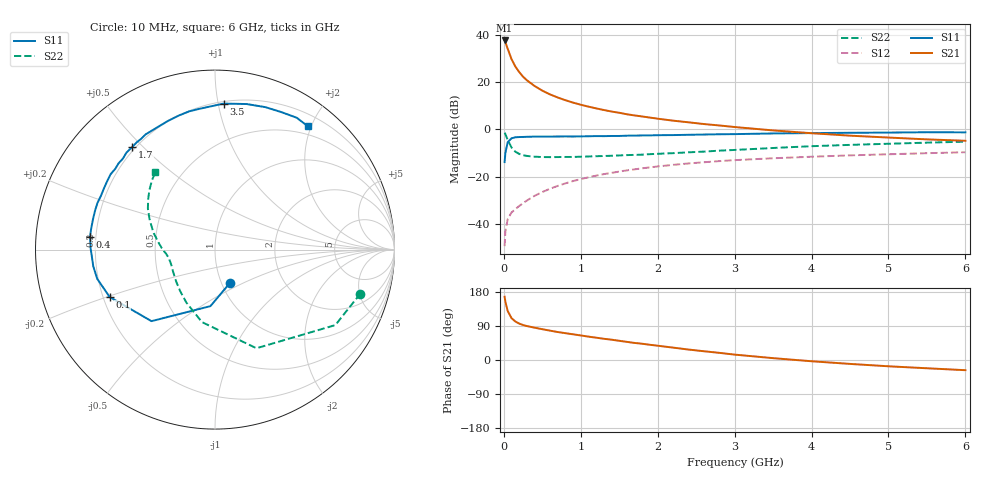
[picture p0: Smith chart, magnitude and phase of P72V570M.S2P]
! SIEMENS Small Signal Semiconductors
! BFP196
! Si NPN RF Bipolar Junction Transistor in SOT143
! VCE = 2.5 V  IC = 70 mA
! Common Emitter S-Parameters:  May  1996
# GHz  S  MA  R  50
!  f  S11  S21  S12  S22
! GHz  MAG  ANG  MAG  ANG  MAG  ANG  MAG  ANG
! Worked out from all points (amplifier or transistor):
!   36 points, 10 MHz to 6 GHz, reference 50 ohm
!   highest |S21| = 37.5 dB at 10 MHz (marker M1)
!   |S21| within 3 dB of that: start of sweep to 44.55 MHz
!   unconditionally stable (mu >= 1): 373.3 MHz to 4.492 GHz
!   at 250 MHz: K = 0.92, MSG = 26.7 dB, |S12| = -31.2 dB
!   at 1.4 GHz: K = 1.09, MAG = 11.1 dB, |S12| = -18.4 dB
!   at 6 GHz: K = 0.99, MSG = 2.4 dB, |S12| = -9.7 dB
!   S11 on the Smith chart (normalised r, x): 10 MHz: 1.10, -0.42; 100 MHz: 0.23, -0.20; 400 MHz: 0.18, +0.05; 1.7 GHz: 0.19, +0.46; 3.5 GHz: 0.21, +1.04; 6 GHz: 0.37, +1.95
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0.01  0.2024 -65.2  74.92 166.9  0.0034 77.6  0.8465 -16.8
0.02  0.3159 -94.6  69.35 153.9  0.007 69.7  0.7914 -32.1
0.05  0.5331 -131.6  49.97 129.3  0.0126 54.3  0.5962 -67.2
0.1  0.6437 -155.8  30.19 110.4  0.0175 49.4  0.4104 -100.2
0.15  0.6761 -166.1  21.05 101.5  0.0206 52.5  0.3354 -118.4
0.2  0.6846 -172.2  16.09 96.1  0.024 56.1  0.3014 -130.2
0.25  0.6876 -177.1  12.86 92.3  0.0274 58.2  0.2828 -138.9
0.3  0.6925 179.8  10.8 89.6  0.0313 61.3  0.2734 -144.6
0.4  0.6996 174.1  8.169 85.2  0.0394 63.8  0.2633 -152.9
0.5  0.6998 170.2  6.53 81.3  0.0472 64.8  0.2588 -158.4
0.6  0.7007 165.7  5.445 77.5  0.0555 65.0  0.2579 -162.1
0.7  0.7028 161.7  4.684 73.8  0.0636 65.2  0.2586 -164.7
0.9  0.7027 154.7  3.649 67.8  0.0806 63.4  0.2601 -169.1
1.1  0.7113 147.7  3.003 61.7  0.0966 61.5  0.2664 -172.0
1.3  0.7152 141.0  2.547 56.0  0.1129 58.9  0.2725 -174.8
1.7  0.7345 129.0  1.956 45.0  0.1424 53.1  0.2876 -179.8
2.2  0.7529 115.7  1.518 32.7  0.1771 45.6  0.3128 174.0
3  0.7893 96.2  1.114 14.2  0.2227 33.4  0.3656 162.2
3.5  0.815 86.6  0.945 4.9  0.2441 26.4  0.4021 155.1
4.5  0.8419 70.5  0.732 -10.3  0.2808 14.3  0.4678 142.7
5.5  0.8644 58.2  0.611 -21.8  0.3123 3.4  0.5214 132.4
6  0.86 52.9  0.571 -26.9  0.3273 -2.3  0.5463 127.4
